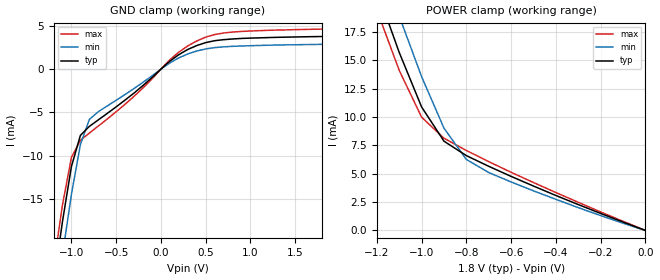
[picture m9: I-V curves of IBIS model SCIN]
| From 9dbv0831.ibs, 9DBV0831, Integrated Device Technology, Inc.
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| Done update up to here
|   Model SCIN
[Model]   SCIN
Model_type   Input
Vinl =   0.54V
Vinh =   1.26V
C_comp   3.40pF   2.85pF   3.95pF
[Temperature Range]   25.00   70.00   0.000
[Voltage Range]   1.80V   1.62V   1.98V
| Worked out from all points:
|   GND clamp passes 1 mA (typ) near -0.10 V on its own axis
|   POWER clamp passes 1 mA (typ) near -0.13 V on its own axis
[GND_clamp]
| voltage   I(typ)   I(min)   I(max)
-1.8V     -72.89mA   -76.87mA   -70.76mA
-1.2V     -24.92mA   -29.01mA   -22.79mA
-1.1V     -17.6mA    -21.48mA   -15.68mA
-1V       -11.25mA   -14.47mA   -10.2mA
-900mV    -7.66mA    -8.72mA    -8.23mA
-800mV    -6.62mA    -5.82mA    -7.39mA
-300mV    -2.76mA    -2.24mA    -3.14mA
100mV     920uA      720uA      1.08mA
300mV     2.27mA     1.75mA     2.68mA
600mV     3.28mA     2.48mA     3.99mA
900mV     3.54mA     2.67mA     4.35mA
1.8V      3.76mA     2.86mA     4.62mA
[POWER_clamp]
| voltage   I(typ)   I(min)   I(max)
-1.8V     57.31mA    60.73mA    55.47mA
-1.2V     21.16mA    24.54mA    19.4mA
-1.1V     15.67mA    18.87mA    14.09mA
-1V       10.87mA    13.54mA    9.97mA
-900mV    7.86mA     9mA        8.12mA
-800mV    6.59mA     6.25mA     7.04mA
-700mV    5.65mA     5.1mA      6.06mA
-600mV    4.76mA     4.27mA     5.12mA
-300mV    2.28mA     2.01mA     2.48mA
0V        44.83pA    370pA      23.45pA
